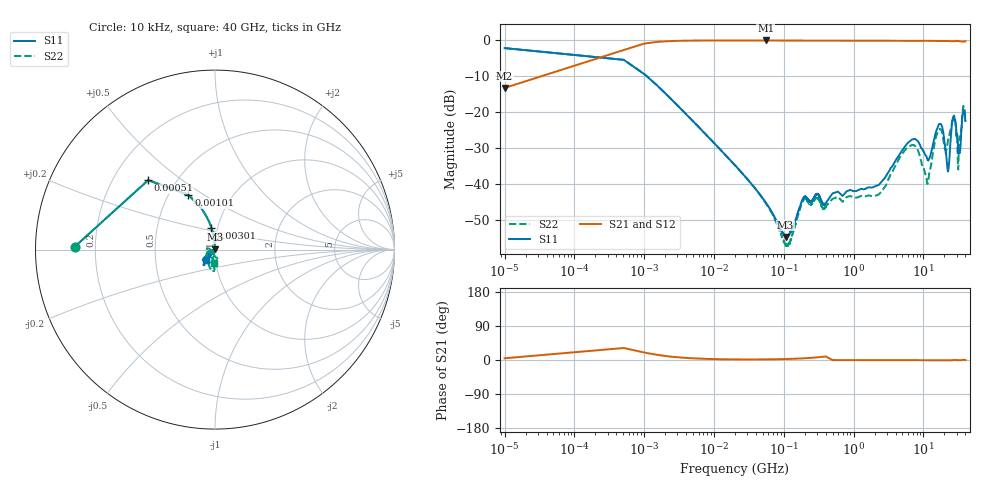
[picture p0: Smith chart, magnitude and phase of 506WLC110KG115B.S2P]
!  American Technical Ceramics  Date:  3/15/2011
!  One Norden Lane
!  Huntington Station,  NY.  11746-2102
!  Tel:  (631) 622-4700  Fax:  (631) 622-4748
!  Part Number  506WLC110KT115B
!  Description:  Ultra-Broadband Inductor
!  Application:  Ultra-broadband DC block decoupling, bias tee
# GHZ S DB R 50
! Freq  |S11|  S11 Ph  |S21|  S21 Ph  |S12|  S12 Ph  |S22|  S22 Ph
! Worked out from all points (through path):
!   1201 points, 10 kHz to 40 GHz, reference 50 ohm
!   highest |S21| = -0.01 dB at 55.01 MHz (marker M1); lowest = -13.2 dB at 10 kHz (marker M2)
!   lowest |S11| = -54.7 dB at 106 MHz (marker M3), VSWR 1.00, Z = 49.8 + j0.0598 ohm
!   |S11| at or under -10 dB: 1.107 MHz to end of sweep
!   |S22| runs from -57.3 to -2.1 dB; largest |S21 - S12| = 0.0024
!   S11 on the Smith chart (normalised r, x): 10 kHz: 0.12, +0.01; 510 kHz: 0.35, +0.38; 1.01 MHz: 0.63, +0.43; 3.01 MHz: 0.93, +0.23; 40 GHz: 0.90, -0.10
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1e-05  -2.13 178.8  -13.22 4.6  -13.25 4.6  -2.13 178.9
0.00051  -5.41 133.9  -2.66 31.7  -2.65 31.6  -5.39 133.9
0.00101  -9.41 115.9  -0.87 19.7  -0.86 19.6  -9.41 115.8
0.00201  -14.74 103.8  -0.24 10.6  -0.24 10.6  -14.74 103.6
0.00301  -18.11 99.5  -0.11 7.2  -0.11 7.2  -18.11 99.2
0.02001  -34.75 94.8  -0.01 1.5  -0.01 1.5  -34.76 92.8
0.05501  -45.12 105.0  -0.01 1.6  -0.01 1.6  -45.24 98.8
0.10601  -54.71 161.0  -0.01 2.5  -0.01 2.5  -56.88 151.8
0.19051  -43.88 -153.9  -0.05 4.3  -0.05 4.3  -44.41 -160.6
0.252  -44.69 -164.9  -0.05 5.8  -0.05 5.9  -45.48 -171.2
3.271  -36.18 -142.5  -0.10 -0.5  -0.09 -0.5  -38.05 -136.4
7.033  -27.53 -129.3  -0.13 -0.4  -0.13 -0.5  -29.08 -109.3
11.587  -33.41 -153.8  -0.09 -0.6  -0.10 -0.6  -39.78 -134.9
17.329  -23.24 -126.6  -0.15 -0.6  -0.15 -0.7  -24.67 -100.2
20.695  -30.44 -135.0  -0.15 -0.7  -0.16 -0.8  -30.51 -132.6
22.576  -36.49 -141.0  -0.18 -0.9  -0.19 -0.9  -27.80 -163.5
26.734  -21.29 -134.0  -0.24 -0.3  -0.25 -0.3  -21.95 -105.0
28.912  -22.77 -143.5  -0.21 0.0  -0.21 -0.0  -23.64 -84.4
31.486  -30.56 -163.3  -0.17 -0.4  -0.17 -0.5  -35.73 -155.1
33.466  -30.63 -162.9  -0.22 -0.5  -0.22 -0.5  -26.77 174.8
36.931  -20.17 -126.3  -0.29 0.4  -0.29 0.4  -18.79 -101.4
40  -22.41 -131.0  -0.24 -0.2  -0.25 -0.2  -22.55 -93.9
